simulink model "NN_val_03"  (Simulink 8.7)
settings: Solver=ode45  StartTime=0.0  StopTime=1000  RelTol=1e-3
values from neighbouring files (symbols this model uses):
  Ts = 0.05    [init_model.m]
libraries: neural x26

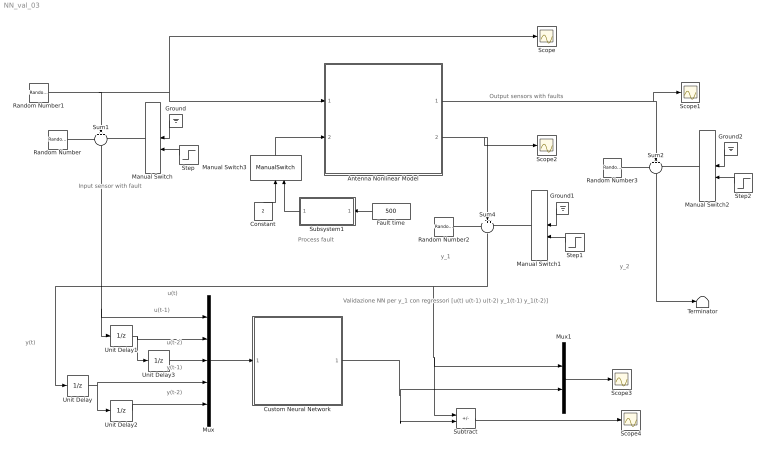
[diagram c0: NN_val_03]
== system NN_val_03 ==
  note: Validazione NN per y_1 con regressori [u(t) u(t-1) u(t-2) y_1(t-1) y_1(t-2)]
  note: y(t)
  note: y(t-1)
  note: y_2
  note: y_1
  note: u(t)
  note: Output sensors with faults
  note: Process fault
  note: Input sensor with fault
  note: u(t-1)
  note: y(t-2)
  note: u(t-2)
  Antenna Nonlinear Model : Subsystem
  Constant : Constant  Value=2
  Custom Neural Network : Subsystem
  Fault time : Constant  Value=500
  Ground : Ground
  Ground1 : Ground
  Ground2 : Ground
  Manual Switch{,1..3} (4 alike) : ManualSwitch
  Mux : Mux  Inputs=5
  Mux1 : Mux  Inputs=2
  Random Number : RandomNumber  Variance=0.0001  Seed=1  SampleTime=Ts
  Random Number1 : RandomNumber  Variance=0.1  SampleTime=10
  Random Number2 : RandomNumber  Variance=0.00001  Seed=2  SampleTime=Ts
  Random Number3 : RandomNumber  Variance=0.00001  Seed=3  SampleTime=Ts
  Scope{,1..4} (5 alike) : Scope
  Step : Step  Time=500  SampleTime=0
  Step1 : Step  Time=1500  SampleTime=0
  Step2 : Step  Time=500  SampleTime=0
  Subsystem1 : Subsystem
  Subtract : Sum  Inputs=+-
  Sum1 : Sum  Inputs=+++  SaturateOnIntegerOverflow=on
  Sum2 : Sum  Inputs=+++  SaturateOnIntegerOverflow=on
  Sum4 : Sum  Inputs=+++  SaturateOnIntegerOverflow=on
  Terminator : Terminator
  Unit Delay{,1..3} (4 alike) : UnitDelay  SampleTime=Ts  HasFrameUpgradeWarning=on
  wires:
  Random Number1/1 -> Scope/1, Antenna Nonlinear Model/1(force), Sum1/2
  Random Number/1 -> Sum1/1
  Manual Switch/1 -> Sum1/3
  Sum1/1 -> Unit Delay1/1, Mux/1
  Ground/1 -> Manual Switch/1
  Step/1 -> Manual Switch/2
  Random Number2/1 -> Sum4/1
  Ground1/1 -> Manual Switch1/1
  Manual Switch1/1 -> Sum4/3
  Step1/1 -> Manual Switch1/2
  Antenna Nonlinear Model/2(velocity) -> Sum4/2, Scope2/1
  Random Number3/1 -> Sum2/1
  Ground2/1 -> Manual Switch2/1
  Manual Switch2/1 -> Sum2/3
  Step2/1 -> Manual Switch2/2
  Antenna Nonlinear Model/1(angle) -> Sum2/2, Scope1/1
  Sum2/1 -> Terminator/1
  Fault time/1 -> Subsystem1/1(Fault time)
  Subsystem1/1(Fault) -> Manual Switch3/2
  Manual Switch3/1 -> Antenna Nonlinear Model/2(drag)
  Constant/1 -> Manual Switch3/1
  Mux/1 -> Custom Neural Network/1(Input)
  Unit Delay/1 -> Mux/4, Unit Delay2/1
  Unit Delay1/1 -> Unit Delay3/1, Mux/2
  Unit Delay3/1 -> Mux/3
  Unit Delay2/1 -> Mux/5
  Custom Neural Network/1(Output) -> Subtract/2, Mux1/2
  Sum4/1 -> Subtract/1, Mux1/1, Unit Delay/1
  Subtract/1 -> Scope4/1
  Mux1/1 -> Scope3/1

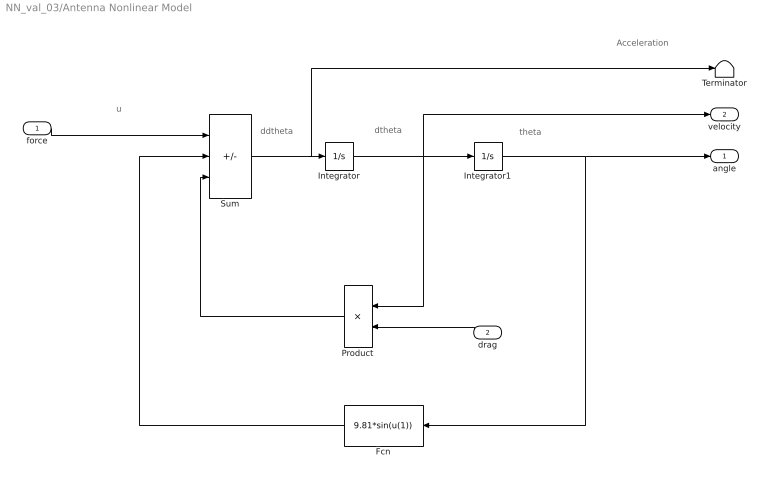
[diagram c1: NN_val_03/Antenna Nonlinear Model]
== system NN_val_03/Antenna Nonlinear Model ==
  note: Acceleration
  note: ddtheta
  note: dtheta
  note: theta
  note: u
  force : Inport
  drag : Inport  Port=2
  Fcn : Fcn  Expr=9.81*sin(u(1))
  Integrator : Integrator
  Integrator1 : Integrator  InitialCondition=(pi/180)*90
  Product : Product
  Sum : Sum  Inputs=+--  SaturateOnIntegerOverflow=on
  Terminator : Terminator
  angle : Outport
  velocity : Outport  Port=2
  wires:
  Sum/1 -> Terminator/1, Integrator/1
  Integrator/1 -> Product/1, Integrator1/1, velocity/1
  Integrator1/1 -> angle/1, Fcn/1
  Fcn/1 -> Sum/2
  Product/1 -> Sum/3
  force/1 -> Sum/1
  drag/1 -> Product/2

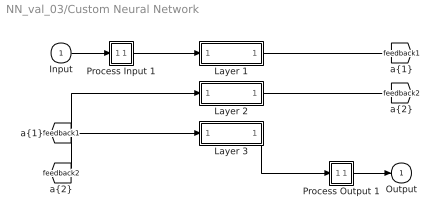
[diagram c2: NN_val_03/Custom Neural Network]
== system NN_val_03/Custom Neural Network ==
  Input : Inport  PortDimensions=5  SampleTime=0.05
  Layer 1 : Subsystem
  Layer 2 : Subsystem
  Layer 3 : Subsystem
  Process Input 1 : Subsystem
  Process Output 1 : Subsystem
  Output : Outport  InitialOutput=0
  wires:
  Input/1 -> Process Input 1/1(x)
  Process Output 1/1(y) -> Output/1
  Process Input 1/1(p) -> Layer 1/1("p{1}")
  Layer 1/1("a{1}") -> [feedback1]
  [feedback1] -> Layer 2/1("a{1} ")
  Layer 2/1("a{2}") -> [feedback2]
  [feedback2] -> Layer 3/1("a{2} ")
  Layer 3/1("a{3}") -> Process Output 1/1(a)

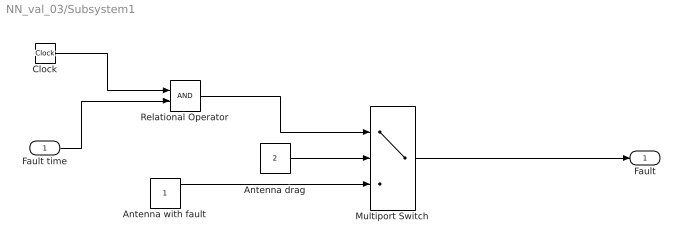
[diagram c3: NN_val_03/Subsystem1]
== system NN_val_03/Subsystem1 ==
  Fault time : Inport
  Antenna drag : Constant  Value=2
  Antenna with fault : Constant
  Clock : Clock
  Multiport Switch : MultiPortSwitch  DataPortOrder=Zero-based contiguous  Inputs=2  zeroidx=on
  Relational Operator : RelationalOperator  OutDataTypeStr=boolean
  Fault : Outport
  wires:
  Clock/1 -> Relational Operator/1
  Fault time/1 -> Relational Operator/2
  Antenna drag/1 -> Multiport Switch/2
  Relational Operator/1 -> Multiport Switch/1
  Multiport Switch/1 -> Fault/1
  Antenna with fault/1 -> Multiport Switch/3

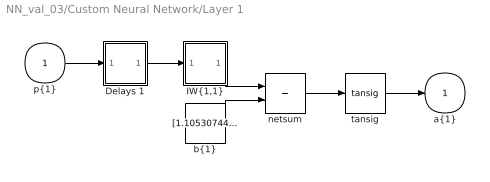
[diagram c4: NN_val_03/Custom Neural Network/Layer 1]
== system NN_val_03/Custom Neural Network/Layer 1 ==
  "p{1}" : Inport  PortDimensions=5  SampleTime=0.05
  Delays 1 : Subsystem
  "IW{1,1}" : Subsystem
  "b{1}" : Constant  Value=[1.10530744380455558939502225257456302642822265625;-0.91987205176696107411515868079732172191143035888671875;0.70121842304207671059401718594017438590526580810546875;-0.91141506916244108271740742566180415451526641845703125;-0.455247033173167447994700296476366929709911346435546875;1.2909449640263073177948172087781131267547607421875;-1.3198955795841964544479196774773299694061279296875]
  netsum : Sum  Inputs=2  InputSameDT=on  SaturateOnIntegerOverflow=on
  tansig : neural/Transfer Functions/tansig
  "a{1}" : Outport  InitialOutput=[0;0;0;0;0;0;0]
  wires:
  "p{1}"/1 -> Delays 1/1("p{1}")
  Delays 1/1("pd{1,1}") -> "IW{1,1}"/1("pd{1,1}")
  "IW{1,1}"/1("iz{1,1}") -> netsum/1
  "b{1}"/1 -> netsum/2
  netsum/1 -> tansig/1
  tansig/1 -> "a{1}"/1

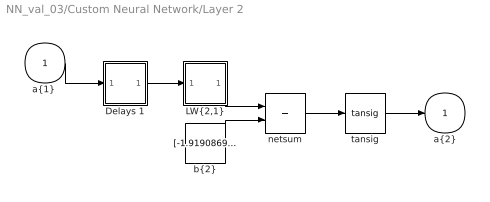
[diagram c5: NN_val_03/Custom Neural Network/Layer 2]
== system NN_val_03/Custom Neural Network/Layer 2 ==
  "a{1} " : Inport  PortDimensions=7  SampleTime=0.05
  Delays 1 : Subsystem
  "LW{2,1}" : Subsystem
  "b{2}" : Constant  Value=[-1.919086920864990997159793550963513553142547607421875;-1.61527237698411330057979284902103245258331298828125;1.4113275257878139523626259688171558082103729248046875;-1.0560270550590988847261542105115950107574462890625;0.85966763486457320464495523992809467017650604248046875;-0.4535197548296887593011206263327039778232574462890625;-0.6674192983500593090440133892116136848926544189453125;0.078559266461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
  netsum : Sum  Inputs=2  InputSameDT=on  SaturateOnIntegerOverflow=on
  tansig : neural/Transfer Functions/tansig
  "a{2}" : Outport  InitialOutput=[0;0;0;0;0;0;0;0;0;0;0;0;0;0;0]
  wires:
  "a{1} "/1 -> Delays 1/1("p{2}")
  Delays 1/1("pd{2,1}") -> "LW{2,1}"/1("ad{2,1}")
  "LW{2,1}"/1("lz{2,1}") -> netsum/1
  "b{2}"/1 -> netsum/2
  netsum/1 -> tansig/1
  tansig/1 -> "a{2}"/1

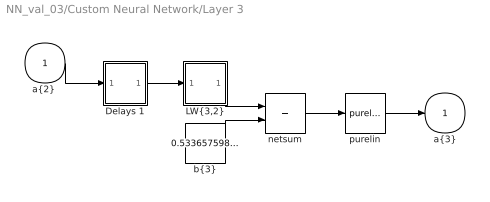
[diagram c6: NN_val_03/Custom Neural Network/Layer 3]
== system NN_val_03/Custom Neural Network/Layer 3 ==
  "a{2} " : Inport  PortDimensions=15  SampleTime=0.05
  Delays 1 : Subsystem
  "LW{3,2}" : Subsystem
  "b{3}" : Constant  Value=0.53365759810026691667417253484018146991729736328125
  netsum : Sum  Inputs=2  InputSameDT=on  SaturateOnIntegerOverflow=on
  purelin : neural/Transfer Functions/purelin
  "a{3}" : Outport  InitialOutput=0
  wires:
  "a{2} "/1 -> Delays 1/1("p{3}")
  Delays 1/1("pd{3,2}") -> "LW{3,2}"/1("ad{3,2}")
  "LW{3,2}"/1("lz{3,2}") -> netsum/1
  "b{3}"/1 -> netsum/2
  netsum/1 -> purelin/1
  purelin/1 -> "a{3}"/1

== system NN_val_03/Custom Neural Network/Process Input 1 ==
  x : Inport  PortDimensions=5  SampleTime=0.05
  p : Outport  PortDimensions=5  SampleTime=0.05
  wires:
  x/1 -> p/1

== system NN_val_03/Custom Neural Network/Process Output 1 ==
  a : Inport  PortDimensions=1  SampleTime=0.05
  y : Outport  PortDimensions=1  SampleTime=0.05
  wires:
  a/1 -> y/1

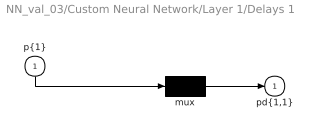
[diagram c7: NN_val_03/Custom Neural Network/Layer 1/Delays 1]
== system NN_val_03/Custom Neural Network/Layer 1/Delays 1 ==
  "p{1}" : Inport  PortDimensions=5  SampleTime=0.05
  mux : Mux  Inputs=1
  "pd{1,1}" : Outport
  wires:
  "p{1}"/1 -> mux/1
  mux/1 -> "pd{1,1}"/1

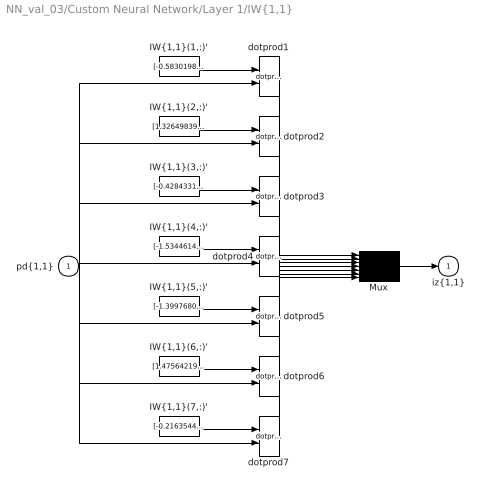
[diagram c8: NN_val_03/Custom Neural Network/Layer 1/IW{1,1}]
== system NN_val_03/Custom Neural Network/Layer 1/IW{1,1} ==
  "pd{1,1}" : Inport  PortDimensions=5  SampleTime=0.05
  "IW{1,1}(1,:)'" : Constant  Value=[-0.583019801330284082041544024832546710968017578125;-1.25508140900980347254289881675504148006439208984375;-1.057440791846882888194159022532403469085693359375;0.628191541881931936330829557846300303936004638671875;-0.6802641997588751987535715670674107968807220458984375]
  "IW{1,1}(2,:)'" : Constant  Value=[1.326498399350281687247843365184962749481201171875;-1.0637199238880994389688794399262405931949615478515625;1.15313512834890463665260540437884628772735595703125;0.052187064969599440689140834592762985266745090484619140625;0.64695368613661441425932707716128788888454437255859375]
  "IW{1,1}(3,:)'" : Constant  Value=[-0.42843316958482569045685295350267551839351654052734375;0.354170149937899025882614978399942629039287567138671875;-1.52671760301469827680875823716633021831512451171875;0.60313164559242149476148142639431171119213104248046875;-0.559821808989564129177551876637153327465057373046875]
  "IW{1,1}(4,:)'" : Constant  Value=[-1.5344614301815131529593827508506365120410919189453125;-1.097932790296682892261515007703565061092376708984375;-0.71910973970002622923658464060281403362751007080078125;0.0785840504264594397199061859282664954662322998046875;-0.6512649664335230514922159272828139364719390869140625]
  "IW{1,1}(5,:)'" : Constant  Value=[-1.3997680162787526914058844340615905821323394775390625;1.1111703843173519334897036969778127968311309814453125;-1.2343280366773239364874825696460902690887451171875;0.68182201005407117033740860279067419469356536865234375;0.38078045549280281623083510567084886133670806884765625]
  "IW{1,1}(6,:)'" : Constant  Value=[1.47564219404607666064066506805829703807830810546875;-1.31289951791481573906139601604081690311431884765625;0.89405414079453471298819522417034022510051727294921875;1.02937116888288660021544274059124290943145751953125;-0.269868547493541388604398889583535492420196533203125]
  "IW{1,1}(7,:)'" : Constant  Value=[-0.216354488200101335859670825811917893588542938232421875;1.5296743484134032176058326513157226145267486572265625;0.8823191112941584091089453067979775369167327880859375;0.60015992551647612263110431740642525255680084228515625;-0.356237495969262740747041107169934548437595367431640625]
  Mux : Mux  Inputs=7
  dotprod{1..7} (7 alike) : neural/Weight Functions/dotprod
  "iz{1,1}" : Outport
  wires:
  "IW{1,1}(1,:)'"/1 -> dotprod1/1
  "pd{1,1}"/1 -> dotprod1/2, dotprod2/2, dotprod3/2, dotprod4/2, dotprod5/2, dotprod6/2, dotprod7/2
  dotprod1/1 -> Mux/1
  "IW{1,1}(2,:)'"/1 -> dotprod2/1
  dotprod2/1 -> Mux/2
  "IW{1,1}(3,:)'"/1 -> dotprod3/1
  dotprod3/1 -> Mux/3
  "IW{1,1}(4,:)'"/1 -> dotprod4/1
  dotprod4/1 -> Mux/4
  "IW{1,1}(5,:)'"/1 -> dotprod5/1
  dotprod5/1 -> Mux/5
  "IW{1,1}(6,:)'"/1 -> dotprod6/1
  dotprod6/1 -> Mux/6
  "IW{1,1}(7,:)'"/1 -> dotprod7/1
  dotprod7/1 -> Mux/7
  Mux/1 -> "iz{1,1}"/1

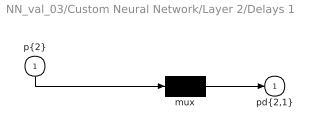
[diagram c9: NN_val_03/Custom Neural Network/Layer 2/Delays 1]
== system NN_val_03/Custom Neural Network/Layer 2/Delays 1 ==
  "p{2}" : Inport  PortDimensions=7  SampleTime=0.05
  mux : Mux  Inputs=1
  "pd{2,1}" : Outport
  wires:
  "p{2}"/1 -> mux/1
  mux/1 -> "pd{2,1}"/1

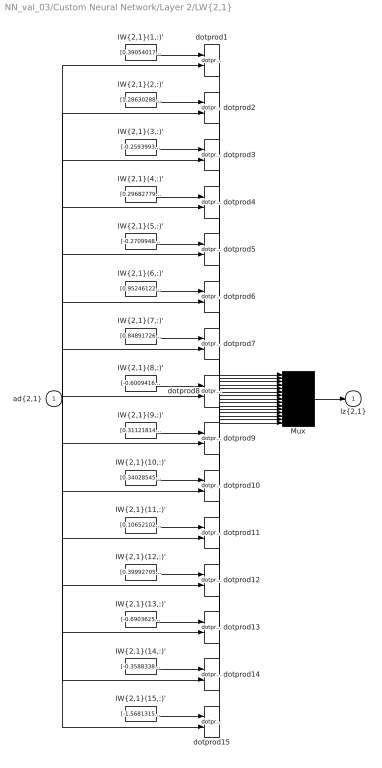
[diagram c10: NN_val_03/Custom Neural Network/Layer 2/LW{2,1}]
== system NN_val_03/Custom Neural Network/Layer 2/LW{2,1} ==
  "ad{2,1}" : Inport  PortDimensions=7  SampleTime=0.05
  "IW{2,1}(1,:)'" : Constant  Value=[0.39054017381308991918587025793385691940784454345703125;1.2575845907471630003016116461367346346378326416015625;-0.1763366642268466844001295612542890012264251708984375;-0.424881015579474163867956804097048006951808929443359375;-0.499728528242604330689147218436119146645069122314453125;1.0119387869523392975423803363810293376445770263671875;1.31781569794268182960195190389640629291534423828125]
  "IW{2,1}(10,:)'" : Constant  Value=[0.3402854583309971037152763528865762054920196533203125;1.2711928959056557619788918600534088909626007080078125;0.52348647073922494055153720182715915143489837646484375;0.570240217662213666471870965324342250823974609375;0.49220605375832937600222294349805451929569244384765625;1.1670253474267671123243417241610586643218994140625;-0.199099340059623430843060987172066234052181243896484375]
  "IW{2,1}(11,:)'" : Constant  Value=[0.106521029979073700300062910173437558114528656005859375;-0.75012261657439449624718008635682053864002227783203125;-1.1460505148686161991378185120993293821811676025390625;-0.75328643767106229223173841091920621693134307861328125;-0.156347536404986831026775462305522523820400238037109375;0.68667939066603855824411084540770389139652252197265625;-1.1024135733470228348807040674728341400623321533203125]
  "IW{2,1}(12,:)'" : Constant  Value=[0.39992705050142074441055228817276656627655029296875;-0.842126884305364864502507771248929202556610107421875;0.17411392349929466494273810894810594618320465087890625;-0.102754537184867100751972657235455699265003204345703125;0.995719287378311168623667981592006981372833251953125;-0.8341091843093251245733199539245106279850006103515625;-0.5463628583168900210154106389381922781467437744140625]
  "IW{2,1}(13,:)'" : Constant  Value=[-0.6903625465470912825338700713473372161388397216796875;-1.0992392663604626523721208286588080227375030517578125;-0.04687877296661734083382810922557837329804897308349609375;0.04706705235039286561171678613391122780740261077880859375;-0.6064425109566162763741203889367170631885528564453125;0.83739731035321363084023005285416729748249053955078125;-1.0640793178925918027744046412408351898193359375]
  "IW{2,1}(14,:)'" : Constant  Value=[-0.358833896455281242676704778205021284520626068115234375;-0.66981715876863068270807843873626552522182464599609375;0.2537524883421269361605254744063131511211395263671875;-0.6125114044476254182569618933484889566898345947265625;0.280632170029646188513794413665891624987125396728515625;1.3430449815924365708497134619392454624176025390625;0.374809964674626849845395781812840141355991363525390625]
  "IW{2,1}(15,:)'" : Constant  Value=[-1.5681315732480218816391470681992359459400177001953125;-0.411032408641479107824778793656150810420513153076171875;-0.05705615596811040857172514506601146422326564788818359375;1.10986445108745979126751990406773984432220458984375;-0.344712647080742951022358511181664653122425079345703125;-0.01107421081424572566198616385690911556594073772430419921875;-0.041264124873331350928928884513879893347620964050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
  "IW{2,1}(2,:)'" : Constant  Value=[1.2863028834231429176071515030344016849994659423828125;0.485126747088950704966947569118929095566272735595703125;-0.53611343957211021749031942817964591085910797119140625;0.57566631978218418819182033985271118581295013427734375;0.84375806021698906977945853213896043598651885986328125;1.1080219963592223830772809378686361014842987060546875;0.241676539177578586503614133107475936412811279296875]
  "IW{2,1}(3,:)'" : Constant  Value=[-0.259399331273914179885053954421891830861568450927734375;0.054708623816609687484646684652034309692680835723876953125;0.5193835870912817398448169114999473094940185546875;0.9065130216466494861293767826282419264316558837890625;0.57731550478563775641305255703628063201904296875;-0.60126911153086537442646886120201088488101959228515625;-1.465578271920802588823562473407946527004241943359375]
  "IW{2,1}(4,:)'" : Constant  Value=[0.29682779770992551160446737412712536752223968505859375;0.44326555441394288603618178967735730111598968505859375;0.79328656592650281798029254787252284586429595947265625;0.01206559554606394073228425867227997514419257640838623046875;-0.13147435435025534022912552245543338358402252197265625;-1.0641961228620908652686694040312431752681732177734375;-1.16802190020742191478575477958656847476959228515625]
  "IW{2,1}(5,:)'" : Constant  Value=[-0.27099483123222778413463629476609639823436737060546875;0.164776311832462829531920078807161189615726470947265625;0.8392605894455951176524877155316062271595001220703125;-0.4548162194716345307909932671464048326015472412109375;-1.422301652182505815602553411736153066158294677734375;0.8875538988238196314028982669697143137454986572265625;-0.2947933674291529637656594786676578223705291748046875]
  "IW{2,1}(6,:)'" : Constant  Value=[0.95246122139337663359270891305641271173954010009765625;0.11271948920572046060062376682253670878708362579345703125;1.1535736814728299037824399420060217380523681640625;-0.7508857630757843626412295634509064257144927978515625;-0.478993471377681945266857610477018170058727264404296875;0.75065857233262212044877514927065931260585784912109375;0.54307570123924231442202881225966848433017730712890625]
  "IW{2,1}(7,:)'" : Constant  Value=[0.84891726229713093676565449641202576458454132080078125;0.6122780852169480425573055981658399105072021484375;0.8506648508877507897096847955253906548023223876953125;0.131473249982146433989527167796040885150432586669921875;-0.40706362602144230411482794806943275034427642822265625;-0.6494015592593580521452167886309325695037841796875;1.195440436033762043877004543901421129703521728515625]
  "IW{2,1}(8,:)'" : Constant  Value=[-0.6009416853113098699878946717944927513599395751953125;0.58889227730632420776402113915537483990192413330078125;-0.834147536610840401039013158879242837429046630859375;-0.79040947995577681695067440159618854522705078125;-0.7364261815938395461245136175421066582202911376953125;0.656838128378006924634746610536240041255950927734375;0.79512969932819055340900149531080387532711029052734375]
  "IW{2,1}(9,:)'" : Constant  Value=[0.311218146609654577883219417344662360846996307373046875;0.1100664012719076711999122153429198078811168670654296875;-1.1024602660299860357184797976515255868434906005859375;-1.28939218295570245942371911951340734958648681640625;-0.886834854507694725356259368709288537502288818359375;-0.21594060032392892178876309117185883224010467529296875;-0.51197564904671011287717874438385479152202606201171875]
  Mux : Mux  Inputs=15
  dotprod{1..15} (15 alike) : neural/Weight Functions/dotprod
  "lz{2,1}" : Outport
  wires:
  "IW{2,1}(1,:)'"/1 -> dotprod1/1
  "ad{2,1}"/1 -> dotprod1/2, dotprod2/2, dotprod3/2, dotprod4/2, dotprod5/2, dotprod6/2, dotprod7/2, dotprod8/2, dotprod9/2, dotprod10/2, dotprod11/2, dotprod12/2, dotprod13/2, dotprod14/2, dotprod15/2
  dotprod1/1 -> Mux/1
  "IW{2,1}(2,:)'"/1 -> dotprod2/1
  dotprod2/1 -> Mux/2
  "IW{2,1}(3,:)'"/1 -> dotprod3/1
  dotprod3/1 -> Mux/3
  "IW{2,1}(4,:)'"/1 -> dotprod4/1
  dotprod4/1 -> Mux/4
  "IW{2,1}(5,:)'"/1 -> dotprod5/1
  dotprod5/1 -> Mux/5
  "IW{2,1}(6,:)'"/1 -> dotprod6/1
  dotprod6/1 -> Mux/6
  "IW{2,1}(7,:)'"/1 -> dotprod7/1
  dotprod7/1 -> Mux/7
  "IW{2,1}(8,:)'"/1 -> dotprod8/1
  dotprod8/1 -> Mux/8
  "IW{2,1}(9,:)'"/1 -> dotprod9/1
  dotprod9/1 -> Mux/9
  "IW{2,1}(10,:)'"/1 -> dotprod10/1
  dotprod10/1 -> Mux/10
  "IW{2,1}(11,:)'"/1 -> dotprod11/1
  dotprod11/1 -> Mux/11
  "IW{2,1}(12,:)'"/1 -> dotprod12/1
  dotprod12/1 -> Mux/12
  "IW{2,1}(13,:)'"/1 -> dotprod13/1
  dotprod13/1 -> Mux/13
  "IW{2,1}(14,:)'"/1 -> dotprod14/1
  dotprod14/1 -> Mux/14
  "IW{2,1}(15,:)'"/1 -> dotprod15/1
  dotprod15/1 -> Mux/15
  Mux/1 -> "lz{2,1}"/1

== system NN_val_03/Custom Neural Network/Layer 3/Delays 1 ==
  "p{3}" : Inport  PortDimensions=15  SampleTime=0.05
  mux : Mux  Inputs=1
  "pd{3,2}" : Outport
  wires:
  "p{3}"/1 -> mux/1
  mux/1 -> "pd{3,2}"/1

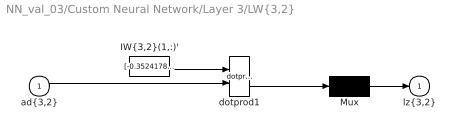
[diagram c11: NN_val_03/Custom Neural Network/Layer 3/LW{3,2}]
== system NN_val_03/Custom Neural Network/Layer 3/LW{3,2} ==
  "ad{3,2}" : Inport  PortDimensions=15  SampleTime=0.05
  "IW{3,2}(1,:)'" : Constant  Value=[-0.35241789578192117549093609341070987284183502197265625;0.321383364243225333467535165254957973957061767578125;-0.57638444986274428583072904075379483401775360107421875;-0.4707125554016589052963581707444973289966583251953125;-0.369934313143426229952837047676439397037029266357421875;0.51660460079753811601932511621271260082721710205078125;0.7161051217893288356464154276181943714618682861328125;-0.078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
  Mux : Mux  Inputs=1
  dotprod1 : neural/Weight Functions/dotprod
  "lz{3,2}" : Outport
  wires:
  "IW{3,2}(1,:)'"/1 -> dotprod1/1
  "ad{3,2}"/1 -> dotprod1/2
  dotprod1/1 -> Mux/1
  Mux/1 -> "lz{3,2}"/1
